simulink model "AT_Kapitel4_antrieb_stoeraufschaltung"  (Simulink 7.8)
settings: Solver=ode15s  StartTime=0.0  StopTime=60  RelTol=1e-3
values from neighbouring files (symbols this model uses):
  c_T = .2e-1    (= 0.02)    [set_data.m]
  d_T = 0    [set_data.m]
  k_A = .9    (= 0.9)    [set_data.m]
  L_A = 3/200    (= 0.015)    [set_data.m]
  R_A = 20    [set_data.m]
  theta_G = .3500000000e-2    (= 0.0035)    [set_data.m]
  theta_L = .6300000000e-2    (= 0.0063)    [set_data.m]
libraries: cstblocks x2

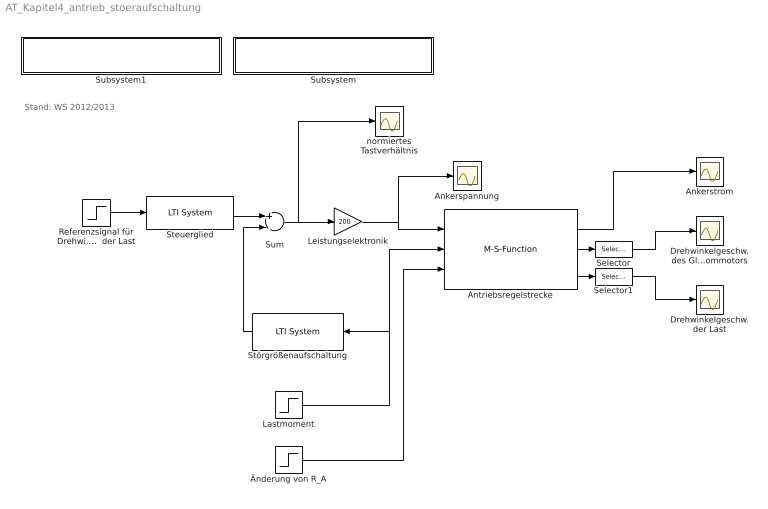
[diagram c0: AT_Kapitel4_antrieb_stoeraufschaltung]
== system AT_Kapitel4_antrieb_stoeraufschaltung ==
  note: Stand: WS 2012/2013
  Ankerspannung : Scope
  Ankerstrom : Scope
  Antriebsregelstrecke : M-S-Function  FunctionName=Antrieb_S_m  Parameters=RAp,LAp,kAp,thetaGp,thetaLp,cTp,dTp  mask{RAp=R_A, LAp=L_A, kAp=k_A, thetaGp=theta_G, thetaLp=theta_L, cTp=c_T, dTp=d_T}
      mask prompts: RAp "Ankerwiderstand"; LAp "Ankerinduktivität"; kAp "Ankerkreiskonstante"; thetaGp "Trägheitsmoment GSM"; thetaLp "Trägheitsmoment Last"; cTp "Federsteifigkeit"; dTp "Dämpfungskonstante"
  Drehwinkelgeschw. der Last : Scope
  Drehwinkelgeschw. des Gleichstrommotors : Scope
  Lastmoment : Step  Time=20  SampleTime=0
  Leistungselektronik : Gain  Gain=200
  Referenzsignal für Drehwinkelgeschw.  der Last : Step  Time=10  Before=100  After=-100  SampleTime=0
  Selector : Selector  InputPortWidth=2  IndexOptions=Index vector (dialog)  Indices=[2]  OutputSizes=1
  Selector1 : Selector  InputPortWidth=2  IndexOptions=Index vector (dialog)  Indices=[2]  OutputSizes=1
  Steuerglied : cstblocks/LTI System  sys=R1  IC=[]
  Störgrößenaufschaltung : cstblocks/LTI System  sys=Rd  IC=[]
  Subsystem : Subsystem  Description=test
  Subsystem1 : Subsystem  Description=test
  Sum : Sum  Inputs=+-
  normiertes Tastverhältnis : Scope
  Änderung von R_A : Step  Time=40  Before=1  After=1.4  SampleTime=0
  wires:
  Leistungselektronik/1 -> Ankerspannung/1, Antriebsregelstrecke/1
  Referenzsignal für Drehwinkelgeschw.  der Last/1 -> Steuerglied/1
  Steuerglied/1 -> Sum/1
  Lastmoment/1 -> Störgrößenaufschaltung/1, Antriebsregelstrecke/2
  Sum/1 -> Leistungselektronik/1, normiertes Tastverhältnis/1
  Störgrößenaufschaltung/1 -> Sum/2
  Änderung von R_A/1 -> Antriebsregelstrecke/3
  Antriebsregelstrecke/1 -> Ankerstrom/1
  Antriebsregelstrecke/2 -> Selector/1
  Selector/1 -> Drehwinkelgeschw. des Gleichstrommotors/1
  Antriebsregelstrecke/3 -> Selector1/1
  Selector1/1 -> Drehwinkelgeschw. der Last/1

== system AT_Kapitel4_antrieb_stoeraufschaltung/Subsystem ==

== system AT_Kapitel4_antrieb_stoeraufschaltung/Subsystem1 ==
